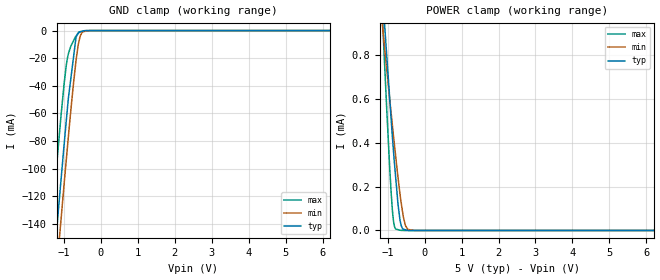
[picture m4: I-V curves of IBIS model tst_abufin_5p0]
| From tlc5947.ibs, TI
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|   tst_abufin_5p0 Model
[Model]   tst_abufin_5p0
Model_type   Input
Vinl = 1.5
Vinh = 3.5
|   typ   min   max
|   (nom PVT)   (Fast PVT)   (slow PVT)
|Average
C_comp   1.289e-12   1.256e-12   1.375e-12
| Where nom  PVT is Nominal Process,  5V,  65C
|   Fast PVT is Strong Process,   5.5V,  -40C
|   Slow PVT is Weak Process,   4.5V,  125C
[Model Spec]
|   typ   min   max
Vinl   1.5   1.35   1.65
Vinh   3.5   3.15   3.85
[Voltage Range]   5   4.5   5.5
|Ambient Temperature   25   85   -40
|Junction Temperature
[Temperature Range]   65   125   -40
[Power Clamp Reference]   5   4.5   5.5
[GND Clamp Reference]   0   0   0
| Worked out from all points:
|   GND clamp passes 1 mA (typ) near -0.57 V on its own axis
|   POWER clamp passes 1 mA (typ) near -1.11 V on its own axis
[GND Clamp]
|   Voltage   I(typ)   I(min)   I(max)
-5V       -1.404A    -1.427A    -1.365A
-1.368V   -199.5mA   -228.3mA   -151.9mA
-1.204V   -147.6mA   -176.5mA   -99.98mA
-1.14V    -127.1mA   -156.2mA   -80.38mA
-1.083V   -109.8mA   -138.7mA   -63.21mA
-990mV    -81.15mA   -109.8mA   -37.42mA
-907.5mV  -57.08mA   -85.23mA   -20.35mA
-675mV    -5.395mA   -22.36mA   -4.093mA
-572mV    -996.7uA   -5.338mA   -843uA
-499.5mV  -482.1uA   -912.4uA   -517.5uA
-315mV    -806.3nA   -5.01uA    -2.763uA
10V       0A         0A         0A
[POWER Clamp]
|   Voltage   I(typ)   I(min)   I(max)
-5V       11.25mA    7.958mA    15.98mA
-1.14V    1.078mA    934.6uA    968.4uA
-1.111V   1.008mA    884.6uA    860.6uA
-1.023V   793.8uA    732.9uA    546.2uA
-902mV    499.7uA    529.2uA    163.9uA
-841.5mV  360.4uA    429.7uA    42.16uA
-781mV    238.2uA    335.8uA    6.421uA
-720mV    119.8uA    241.9uA    3.755uA
-635mV    22.67uA    127.5uA    381nA
-522mV    3.425uA    23.89uA    41nA
-459mV    975.1nA    5.134uA    36.07nA
10V       0A         0A         0A
